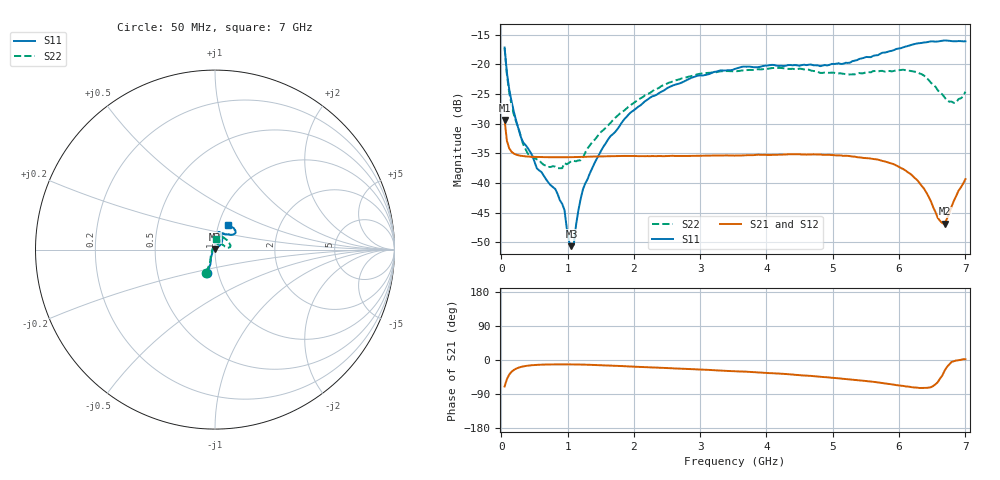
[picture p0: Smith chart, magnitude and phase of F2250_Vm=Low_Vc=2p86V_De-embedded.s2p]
! Integrated Device Technology
! Corporate Headquarters
! 6024 Silver Creek Valley Road
! San Jose, CA 95138  USA
! Phone:  1-408-284-8200
! Toll Free:  1-800-223-1366
! Webpage:  http://www.idt.com/
! Timing and RF Division
! 515 Groton Road, Suite 102
! Westford, MA 01886-6024
! Device:  F2250
! Description: Voltage Variable RF Attenuator
! Frequency:  50.0 -  6000.00 MHz
! Package:  3x3 mm Thin QFN Plastic Package: 16 pin
! Ports:  2 RF, 3 DC
!  Pin  1  = GND
!  Pin  2  = NC
!  Pin  3  = RF1  = Port 1
!  Pin  4  = NC
!  Pin  5  = GND
!  Pin  6  = GND
!  Pin  7  = GND
!  Pin  8  = GND
!  Pin  9  = NC
!  Pin 10  = RF2  = Port 2
!  Pin 11  = NC
!  Pin 12  = GND
!  Pin 13  = GND
!  Pin 14  = VCNTRL
!  Pin 15  = VDD
!  Pin 16  = VMODE
! Vcntrl:  2.860 Volts
! Vmode:  +0.000 Volts
! Vdd:  +3.30  Volts
! Current:  1.175 mA
! Data:  The device was measured on a the F2250 evaluation board which has
!  individual transmission lines to the RF pins.  Data was collected
!  using a calibrated network analyzer.  The evaluation board was
!  de-embedded using a TRL calibration technique.
!  The reference plane is the edge of the package pin.
! Misc:  SN 10
!  Action Tracker AT0258
! Date Measured:  2014-11-26
! Date:  2015-10-15  MJV
! Note:
!  Integrated Device Technology supplies this data as a sample of measured
!  data at the package pin for this product.  Your particular data for this
!  product may vary.
!  Data was taken at 25 degrees C.
!  Integrated Device Technology reserves the right to change this data at anytime.
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# GHz S dB R 50
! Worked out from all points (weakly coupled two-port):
!   201 points, 50 MHz to 7 GHz, reference 50 ohm
!   highest |S21| = -29.42 dB at 50 MHz (marker M1); lowest = -46.9 dB at 6.687 GHz (marker M2)
!   lowest |S11| = -50.7 dB at 1.058 GHz (marker M3), VSWR 1.01, Z = 49.8 + j0.245 ohm
!   |S11| at or under -10 dB: start of sweep to end of sweep
!   |S22| runs from -37.5 to -17.3 dB; largest |S21 - S12| = 6.2e-05
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0.05  -17.18 -108.6  -29.42 -69.8  -29.41 -69.8  -17.28 -111.0
0.08475  -21.45 -107.5  -32.92 -50.3  -32.92 -50.4  -21.75 -110.2
0.15425  -26.23 -116.6  -34.76 -31.1  -34.76 -31.1  -26.81 -122.5
0.29325  -32.22 -127.8  -35.43 -18.5  -35.43 -18.5  -32.10 -137.4
0.3975  -34.09 -141.7  -35.56 -15.0  -35.56 -15.0  -35.04 -160.5
0.91875  -43.55 157.8  -35.69 -11.5  -35.69 -11.5  -37.52 133.4
0.9535  -44.60 170.0  -35.68 -11.5  -35.69 -11.5  -36.66 131.1
1.023  -49.95 143.2  -35.67 -11.6  -35.67 -11.6  -36.62 116.0
1.05775  -50.67 123.0  -35.67 -11.6  -35.67 -11.6  -36.29 110.8
1.0925  -50.47 89.1  -35.66 -11.7  -35.65 -11.7  -36.30 106.2
1.162  -44.67 56.9  -35.64 -11.9  -35.64 -11.9  -36.22 95.4
1.2315  -41.09 44.1  -35.61 -12.1  -35.61 -12.1  -35.79 85.9
1.6485  -32.11 41.9  -35.52 -14.6  -35.52 -14.6  -29.88 64.6
1.96125  -28.04 42.2  -35.46 -17.2  -35.46 -17.2  -26.81 56.8
2.37825  -24.86 47.3  -35.47 -20.3  -35.48 -20.3  -23.99 56.8
3.525  -20.79 72.5  -35.40 -29.5  -35.40 -29.5  -21.19 74.7
4.7065  -20.17 72.3  -35.19 -42.6  -35.19 -42.6  -21.14 72.2
5.85325  -17.81 40.5  -36.63 -63.4  -36.63 -63.5  -21.14 23.0
6.27025  -16.50 40.0  -39.50 -72.9  -39.50 -72.8  -21.36 9.7
6.68725  -16.00 48.7  -46.90 -27.8  -46.87 -27.4  -25.62 28.6
6.861  -16.13 55.1  -42.21 -1.4  -42.17 -1.4  -26.45 57.9
7  -16.13 63.2  -39.37 1.9  -39.33 1.8  -24.62 83.1
